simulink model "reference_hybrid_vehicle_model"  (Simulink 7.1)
settings: Solver=ode3  SolverMode=SingleTasking  StartTime=0.0  StopTime=140  FixedStep=hilsmdl.simulation.stepsize.value  MaxStep=0.01  RelTol=1e-3  AbsTol=1e-3
libraries: HILS_model_library x8

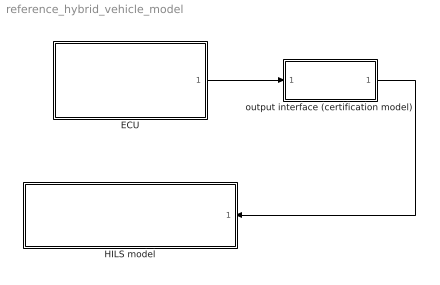
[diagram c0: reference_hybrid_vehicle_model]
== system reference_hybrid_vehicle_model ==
  ECU : Subsystem
  HILS model : Subsystem  Orientation=left
  output interface (certification model) : Subsystem
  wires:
  ECU/1(cmd out) -> output interface (certification model)/1(from ECU)
  output interface (certification model)/1(cmd out) -> HILS model/1(From Ctrl)

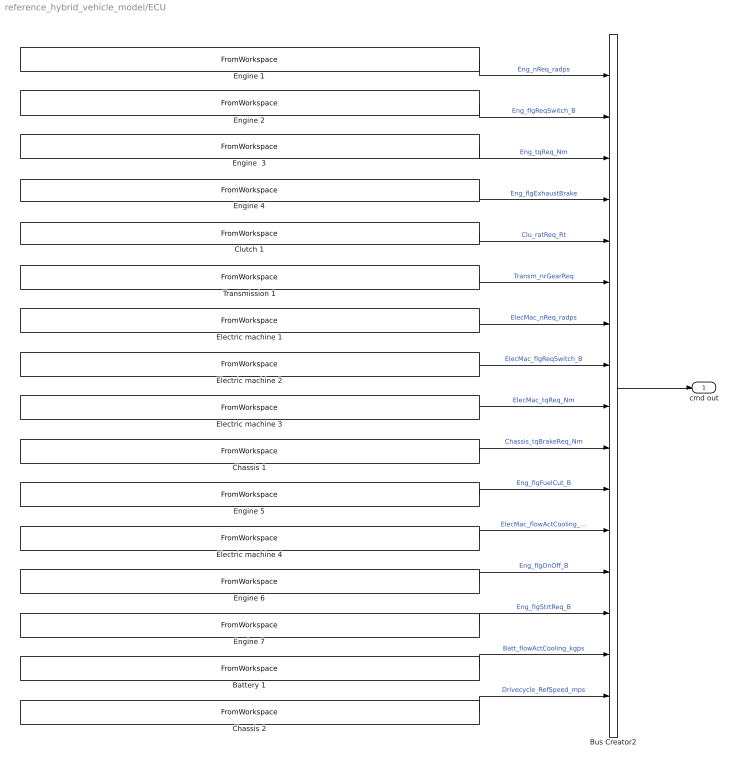
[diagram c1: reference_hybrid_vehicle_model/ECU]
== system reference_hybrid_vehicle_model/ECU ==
  Battery 1 : FromWorkspace  VariableName=[certmdl_input.Batt_flowActCooling_kgps.time.vec,certmdl_input.Batt_flowActCooling_kgps.data.vec]
  Bus Creator2 : BusCreator  Inputs=16
  Chassis 1 : FromWorkspace  VariableName=[certmdl_input.Chassis_tqBrakeReq_Nm.time.vec,certmdl_input.Chassis_tqBrakeReq_Nm.data.vec]
  Chassis 2 : FromWorkspace  VariableName=[hilsmdl.drivecycle.time.vec hilsmdl.drivecycle.speed.vec]
  Clutch 1 : FromWorkspace  VariableName=[certmdl_input.Clu_ratReq_Rt.time.vec,certmdl_input.Clu_ratReq_Rt.data.vec]
  Electric machine 1 : FromWorkspace  VariableName=[certmdl_input.ElecMac_nReq_radps.time.vec,certmdl_input.ElecMac_nReq_radps.data.vec]
  Electric machine 2 : FromWorkspace  VariableName=[certmdl_input.ElecMac_flgReqSwitch_B.time.vec,certmdl_input.ElecMac_flgReqSwitch_B.data.vec]
  Electric machine 3 : FromWorkspace  VariableName=[certmdl_input.ElecMac_tqReq_Nm.time.vec,certmdl_input.ElecMac_tqReq_Nm.data.vec]
  Electric machine 4 : FromWorkspace  VariableName=[certmdl_input.ElecMac_flowActCooling_kgps.time.vec,certmdl_input.ElecMac_flowActCooling_kgps.data.vec]
  Engine  3 : FromWorkspace  VariableName=[certmdl_input.Eng_tqReq_Nm.time.vec,certmdl_input.Eng_tqReq_Nm.data.vec]
  Engine 1 : FromWorkspace  VariableName=[certmdl_input.Eng_nReq_radps.time.vec,certmdl_input.Eng_nReq_radps.data.vec]
  Engine 2 : FromWorkspace  VariableName=[certmdl_input.Eng_flgReqSwitch_B.time.vec,certmdl_input.Eng_flgReqSwitch_B.data.vec]
  Engine 4 : FromWorkspace  VariableName=[certmdl_input.Eng_flgExhaustBrake.time.vec,certmdl_input.Eng_flgExhaustBrake.data.vec]
  Engine 5 : FromWorkspace  VariableName=[certmdl_input.Eng_flgFuelCut_B.time.vec,certmdl_input.Eng_flgFuelCut_B.data.vec]
  Engine 6 : FromWorkspace  VariableName=[certmdl_input.Eng_flgOnOff_B.time.vec,certmdl_input.Eng_flgOnOff_B.data.vec]
  Engine 7 : FromWorkspace  VariableName=[certmdl_input.Eng_flgStrtReq_B.time.vec,certmdl_input.Eng_flgStrtReq_B.data.vec]
  Transmission 1 : FromWorkspace  VariableName=[certmdl_input.Transm_nrGearReq.time.vec,certmdl_input.Transm_nrGearReq.data.vec]
  cmd out : Outport
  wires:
  Bus Creator2/1 -> cmd out/1
  Engine 2/1 -> Bus Creator2/2  "Eng_flgReqSwitch_B"
  Clutch 1/1 -> Bus Creator2/5  "Clu_ratReq_Rt"
  Electric machine 2/1 -> Bus Creator2/8  "ElecMac_flgReqSwitch_B"
  Electric machine 1/1 -> Bus Creator2/7  "ElecMac_nReq_radps"
  Engine 1/1 -> Bus Creator2/1  "Eng_nReq_radps"
  Engine 4/1 -> Bus Creator2/4  "Eng_flgExhaustBrake"
  Engine 5/1 -> Bus Creator2/11  "Eng_flgFuelCut_B"
  Engine 6/1 -> Bus Creator2/13  "Eng_flgOnOff_B"
  Engine 7/1 -> Bus Creator2/14  "Eng_flgStrtReq_B"
  Engine  3/1 -> Bus Creator2/3  "Eng_tqReq_Nm"
  Chassis 1/1 -> Bus Creator2/10  "Chassis_tqBrakeReq_Nm"
  Electric machine 3/1 -> Bus Creator2/9  "ElecMac_tqReq_Nm"
  Transmission 1/1 -> Bus Creator2/6  "Transm_nrGearReq"
  Electric machine 4/1 -> Bus Creator2/12  "ElecMac_flowActCooling_kgps"
  Battery 1/1 -> Bus Creator2/15  "Batt_flowActCooling_kgps"
  Chassis 2/1 -> Bus Creator2/16  "Drivecycle_RefSpeed_mps"

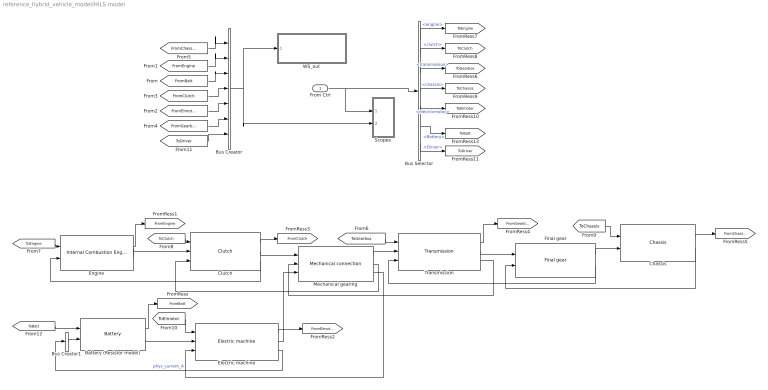
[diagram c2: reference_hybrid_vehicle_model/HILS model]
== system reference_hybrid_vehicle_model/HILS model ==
  From Ctrl : Inport
  Battery (Resistor model) : HILS_model_library/Rechargable energy storage systems/Battery  dat=hilsmdl.battery
  Bus Creator : BusCreator  Inputs=7
  Bus Creator1 : BusCreator  Inputs=1
  Bus Selector : BusSelector  OutputSignals=engine,clutch,transmission,chassis,electricmotor,Battery,Driver
  Chassis : HILS_model_library/Chassis/Chassis  dat=hilsmdl.chassis
  Clutch : HILS_model_library/Mechanical components/Clutch  dat=hilsmdl.clutch
  Electric machine : HILS_model_library/Energy converters/Electric machine  dat=hilsmdl.elmachine
  Engine : HILS_model_library/Energy converters/Internal Combustion Engine  dat=hilsmdl.eng
  Final gear : HILS_model_library/Mechanical components/Final gear  dat=hilsmdl.finalgear
  Mechanical gearing : HILS_model_library/Mechanical components/Mechanical connection  dat=hilsmdl.mechconnection
  Scopes : Subsystem
  Transmission : HILS_model_library/Mechanical components/Transmission  dat=hilsmdl.transmission
  WS_out : Subsystem
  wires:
  Battery (Resistor model)/2 -> Electric machine/2
  Mechanical gearing/3 -> Electric machine/3
  Mechanical gearing/1 -> Transmission/2
  Bus Creator/1 -> Scopes/2(plnt in), WS_out/1(from model)
  Clutch/2 -> Mechanical gearing/1
  Mechanical gearing/2 -> Clutch/3
  Clutch/3 -> Engine/2
  Transmission/3 -> Mechanical gearing/2
  Engine/2 -> Clutch/2
  Chassis/1 -> [FromChassis]
  From Ctrl/1 -> Scopes/1(ctrl in), Bus Selector/1
  Electric machine/2 -> Mechanical gearing/3
  Battery (Resistor model)/1 -> [FromBatt]
  [FromBatt] -> Bus Creator/3
  Engine/1 -> [FromEngine]
  [FromEngine] -> Bus Creator/2
  [FromElmotor] -> Bus Creator/5
  Electric machine/1 -> [FromElmotor]
  [FromClutch] -> Bus Creator/4
  Clutch/1 -> [FromClutch]
  [FromGearbox] -> Bus Creator/6
  Transmission/1 -> [FromGearbox]
  [FromChassis] -> Bus Creator/1
  Bus Selector/3 -> [ToGearbox]  "<transmission>"
  [ToGearbox] -> Transmission/1
  Bus Selector/1 -> [ToEngine]  "<engine>"
  Bus Selector/2 -> [ToClutch]  "<clutch>"
  Bus Selector/4 -> [ToChassis]  "<chassis>"
  Bus Selector/5 -> [ToElmotor]  "<electricmotor>"
  [ToEngine] -> Engine/1
  [ToClutch] -> Clutch/1
  [ToChassis] -> Chassis/1
  [ToElmotor] -> Electric machine/1
  [ToBatt] -> Battery (Resistor model)/1
  Bus Creator1/1 -> Battery (Resistor model)/2
  Electric machine/3 -> Bus Creator1/1  "phys_current_A"
  Transmission/2 -> Final gear/1
  Final gear/2 -> Transmission/3
  Final gear/1 -> Chassis/2
  Chassis/2 -> Final gear/2
  Bus Selector/6 -> [ToBatt]  "<Battery>"
  Bus Selector/7 -> [ToDriver]  "<Driver>"
  [ToDriver] -> Bus Creator/7

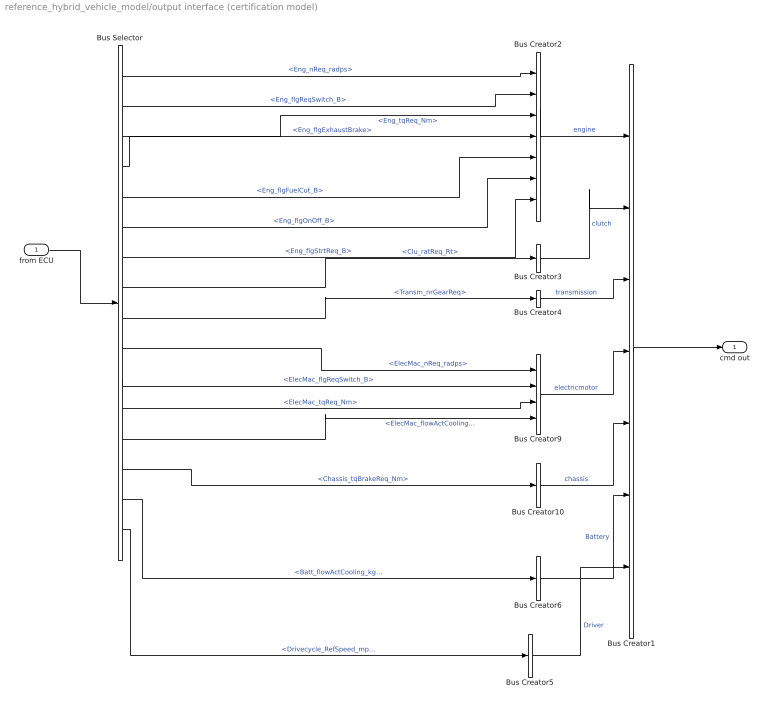
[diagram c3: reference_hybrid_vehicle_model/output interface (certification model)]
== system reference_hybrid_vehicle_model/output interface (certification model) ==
  from ECU : Inport
  Bus Creator1 : BusCreator  Inputs=7
  Bus Creator{3..6,10} (5 alike) : BusCreator  Inputs=1
  Bus Creator2 : BusCreator  Inputs=7
  Bus Creator9 : BusCreator
  Bus Selector : BusSelector  OutputSignals=Eng_nReq_radps,Eng_flgReqSwitch_B,Eng_tqReq_Nm,Eng_flgExhaustBrake,Eng_flgFuelCut_B,Eng_flgOnOff_B,Eng_flgStrtReq_B,Clu_ratReq_Rt,Transm_nrGearReq,ElecMac_nReq_radps,ElecMac_flgReqSwitch_B,ElecMac_tqReq_Nm,ElecMac_flowActCooling_kgps,Chassis_tqBrakeReq_Nm,Batt_flowActCooling_kgps,Drivecycle_RefSpeed_mps
  cmd out : Outport
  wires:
  from ECU/1 -> Bus Selector/1
  Bus Creator4/1 -> Bus Creator1/3  "transmission"
  Bus Creator3/1 -> Bus Creator1/2  "clutch"
  Bus Creator10/1 -> Bus Creator1/5  "chassis"
  Bus Creator9/1 -> Bus Creator1/4  "electricmotor"
  Bus Selector/11 -> Bus Creator9/2  "<ElecMac_flgReqSwitch_B>"
  Bus Selector/10 -> Bus Creator9/1  "<ElecMac_nReq_radps>"
  Bus Creator1/1 -> cmd out/1
  Bus Creator2/1 -> Bus Creator1/1  "engine"
  Bus Selector/1 -> Bus Creator2/1  "<Eng_nReq_radps>"
  Bus Selector/2 -> Bus Creator2/2  "<Eng_flgReqSwitch_B>"
  Bus Selector/3 -> Bus Creator2/3  "<Eng_tqReq_Nm>"
  Bus Selector/12 -> Bus Creator9/3  "<ElecMac_tqReq_Nm>"
  Bus Selector/4 -> Bus Creator2/4  "<Eng_flgExhaustBrake>"
  Bus Selector/8 -> Bus Creator3/1  "<Clu_ratReq_Rt>"
  Bus Selector/9 -> Bus Creator4/1  "<Transm_nrGearReq>"
  Bus Selector/14 -> Bus Creator10/1  "<Chassis_tqBrakeReq_Nm>"
  Bus Selector/5 -> Bus Creator2/5  "<Eng_flgFuelCut_B>"
  Bus Selector/6 -> Bus Creator2/6  "<Eng_flgOnOff_B>"
  Bus Selector/7 -> Bus Creator2/7  "<Eng_flgStrtReq_B>"
  Bus Selector/15 -> Bus Creator6/1  "<Batt_flowActCooling_kgps>"
  Bus Creator6/1 -> Bus Creator1/6  "Battery"
  Bus Selector/13 -> Bus Creator9/4  "<ElecMac_flowActCooling_kgps>"
  Bus Selector/16 -> Bus Creator5/1  "<Drivecycle_RefSpeed_mps>"
  Bus Creator5/1 -> Bus Creator1/7  "Driver"

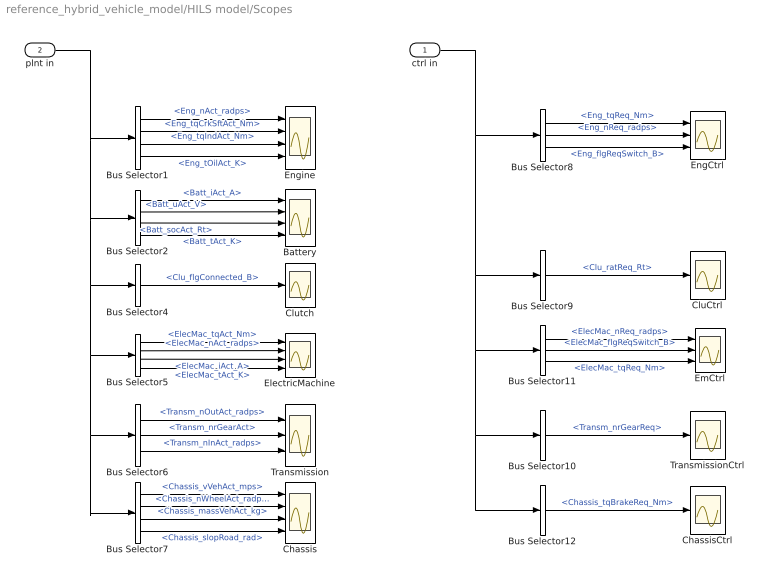
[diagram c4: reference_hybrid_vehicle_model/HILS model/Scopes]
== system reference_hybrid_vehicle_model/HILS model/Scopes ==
  ctrl in : Inport
  plnt in : Inport  Port=2
  Battery : Scope  NumInputPorts=4
  Bus Selector1 : BusSelector  OutputSignals=Engine.Eng_nAct_radps,Engine.Eng_tqCrkSftAct_Nm,Engine.Eng_tqIndAct_Nm,Engine.Eng_tOilAct_K
  Bus Selector10 : BusSelector  OutputSignals=transmission.Transm_nrGearReq
  Bus Selector11 : BusSelector  OutputSignals=electricmotor.ElecMac_nReq_radps,electricmotor.ElecMac_flgReqSwitch_B,electricmotor.ElecMac_tqReq_Nm
  Bus Selector12 : BusSelector  OutputSignals=chassis.Chassis_tqBrakeReq_Nm
  Bus Selector2 : BusSelector  OutputSignals=Battery.Batt_iAct_A,Battery.Batt_uAct_V,Battery.Batt_socAct_Rt,Battery.Batt_tAct_K
  Bus Selector4 : BusSelector  OutputSignals=Clutch.Clu_flgConnected_B
  Bus Selector5 : BusSelector  OutputSignals=ElectricMachine.ElecMac_tqAct_Nm,ElectricMachine.ElecMac_nAct_radps,ElectricMachine.ElecMac_iAct_A,ElectricMachine.ElecMac_tAct_K
  Bus Selector6 : BusSelector  OutputSignals=Transmission.Transm_nOutAct_radps,Transmission.Transm_nrGearAct,Transmission.Transm_nInAct_radps
  Bus Selector7 : BusSelector  OutputSignals=Chassis.Chassis_vVehAct_mps,Chassis.Chassis_nWheelAct_radps,Chassis.Chassis_massVehAct_kg,Chassis.Chassis_slopRoad_rad
  Bus Selector8 : BusSelector  OutputSignals=engine.Eng_tqReq_Nm,engine.Eng_nReq_radps,engine.Eng_flgReqSwitch_B
  Bus Selector9 : BusSelector  OutputSignals=clutch.Clu_ratReq_Rt
  Chassis : Scope  NumInputPorts=4
  ChassisCtrl : Scope
  CluCtrl : Scope
  Clutch : Scope
  ElectricMachine : Scope  NumInputPorts=4
  EmCtrl : Scope  NumInputPorts=3
  EngCtrl : Scope  NumInputPorts=3
  Engine : Scope  NumInputPorts=4
  Transmission : Scope  NumInputPorts=3
  TransmissionCtrl : Scope
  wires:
  plnt in/1 -> Bus Selector1/1, Bus Selector2/1, Bus Selector4/1, Bus Selector5/1, Bus Selector6/1, Bus Selector7/1
  Bus Selector1/1 -> Engine/1  "<Eng_nAct_radps>"
  Bus Selector1/2 -> Engine/2  "<Eng_tqCrkSftAct_Nm>"
  Bus Selector2/1 -> Battery/1  "<Batt_iAct_A>"
  Bus Selector2/2 -> Battery/2  "<Batt_uAct_V>"
  Bus Selector2/3 -> Battery/3  "<Batt_socAct_Rt>"
  Bus Selector4/1 -> Clutch/1  "<Clu_flgConnected_B>"
  Bus Selector5/1 -> ElectricMachine/1  "<ElecMac_tqAct_Nm>"
  Bus Selector5/2 -> ElectricMachine/2  "<ElecMac_nAct_radps>"
  Bus Selector6/1 -> Transmission/1  "<Transm_nOutAct_radps>"
  Bus Selector6/2 -> Transmission/2  "<Transm_nrGearAct>"
  Bus Selector6/3 -> Transmission/3  "<Transm_nInAct_radps>"
  Bus Selector7/1 -> Chassis/1  "<Chassis_vVehAct_mps>"
  Bus Selector7/2 -> Chassis/2  "<Chassis_nWheelAct_radps>"
  Bus Selector7/3 -> Chassis/3  "<Chassis_massVehAct_kg>"
  Bus Selector7/4 -> Chassis/4  "<Chassis_slopRoad_rad>"
  ctrl in/1 -> Bus Selector8/1, Bus Selector9/1, Bus Selector11/1, Bus Selector10/1, Bus Selector12/1
  Bus Selector8/1 -> EngCtrl/1  "<Eng_tqReq_Nm>"
  Bus Selector8/2 -> EngCtrl/2  "<Eng_nReq_radps>"
  Bus Selector9/1 -> CluCtrl/1  "<Clu_ratReq_Rt>"
  Bus Selector10/1 -> TransmissionCtrl/1  "<Transm_nrGearReq>"
  Bus Selector11/1 -> EmCtrl/1  "<ElecMac_nReq_radps>"
  Bus Selector11/2 -> EmCtrl/2  "<ElecMac_flgReqSwitch_B>"
  Bus Selector11/3 -> EmCtrl/3  "<ElecMac_tqReq_Nm>"
  Bus Selector12/1 -> ChassisCtrl/1  "<Chassis_tqBrakeReq_Nm>"
  Bus Selector8/3 -> EngCtrl/3  "<Eng_flgReqSwitch_B>"
  Bus Selector1/3 -> Engine/3  "<Eng_tqIndAct_Nm>"
  Bus Selector1/4 -> Engine/4  "<Eng_tOilAct_K>"
  Bus Selector2/4 -> Battery/4  "<Batt_tAct_K>"
  Bus Selector5/3 -> ElectricMachine/3  "<ElecMac_iAct_A>"
  Bus Selector5/4 -> ElectricMachine/4  "<ElecMac_tAct_K>"

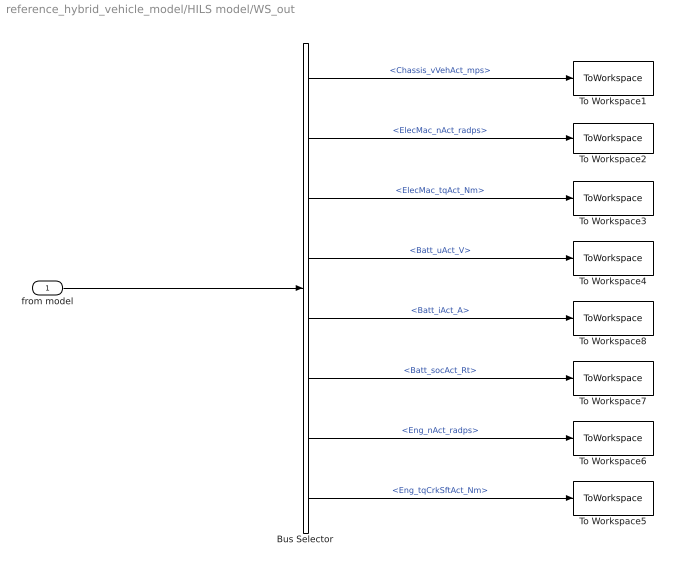
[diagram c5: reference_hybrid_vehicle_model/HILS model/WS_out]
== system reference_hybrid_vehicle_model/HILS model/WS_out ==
  from model : Inport
  Bus Selector : BusSelector  OutputSignals=Chassis.Chassis_vVehAct_mps,ElectricMachine.ElecMac_nAct_radps,ElectricMachine.ElecMac_tqAct_Nm,Battery.Batt_uAct_V,Battery.Batt_iAct_A,Battery.Batt_socAct_Rt,Engine.Eng_nAct_radps,Engine.Eng_tqCrkSftAct_Nm
  To Workspace1 : ToWorkspace  VariableName=Chassis_vVehAct_mps  SampleTime=hilsmdl.simulation.sampletime.value  SaveFormat=Structure With Time
  To Workspace2 : ToWorkspace  VariableName=ElecMac_nAct_radps  SampleTime=hilsmdl.simulation.sampletime.value  SaveFormat=Structure With Time
  To Workspace3 : ToWorkspace  VariableName=ElecMac_tqAct_Nm  SampleTime=hilsmdl.simulation.sampletime.value  SaveFormat=Structure With Time
  To Workspace4 : ToWorkspace  VariableName=Batt_uAct_V  SampleTime=hilsmdl.simulation.sampletime.value  SaveFormat=Structure With Time
  To Workspace5 : ToWorkspace  VariableName=Eng_tqCrkSftAct_Nm  SampleTime=hilsmdl.simulation.sampletime.value  SaveFormat=Structure With Time
  To Workspace6 : ToWorkspace  VariableName=Eng_nAct_radps  SampleTime=hilsmdl.simulation.sampletime.value  SaveFormat=Structure With Time
  To Workspace7 : ToWorkspace  VariableName=Batt_socAct_Rt  SampleTime=hilsmdl.simulation.sampletime.value  SaveFormat=Structure With Time
  To Workspace8 : ToWorkspace  VariableName=Batt_iAct_A  SampleTime=hilsmdl.simulation.sampletime.value  SaveFormat=Structure With Time
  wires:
  from model/1 -> Bus Selector/1
  Bus Selector/1 -> To Workspace1/1  "<Chassis_vVehAct_mps>"
  Bus Selector/2 -> To Workspace2/1  "<ElecMac_nAct_radps>"
  Bus Selector/3 -> To Workspace3/1  "<ElecMac_tqAct_Nm>"
  Bus Selector/4 -> To Workspace4/1  "<Batt_uAct_V>"
  Bus Selector/5 -> To Workspace8/1  "<Batt_iAct_A>"
  Bus Selector/6 -> To Workspace7/1  "<Batt_socAct_Rt>"
  Bus Selector/7 -> To Workspace6/1  "<Eng_nAct_radps>"
  Bus Selector/8 -> To Workspace5/1  "<Eng_tqCrkSftAct_Nm>"
